ORGANIZATION_BLOCK OB 1
	VAR_TEMP
		TMPDUMMY	: INT;
		DTTEMP		: DATE_AND_TIME;
	END_VAR
BEGIN

	// Check forwarding of compound data type to FC
	// (This will create implicit DB pointers)
	AUF		DB 42
	LAR1		P##DTTEMP
	L		DW#16#12345678
	T		D [AR1, P#0.0]
	L		DW#16#87654321
	T		DBD 4
	L		DW#16#AABBCCDD
	T		D [AR1, P#4.0]
	L		DW#16#DDCCBBAA
	T		DBD 8
	CALL		FC 1 (
		DTTEMP	:= #DTTEMP,
		DTDB	:= DB42.DTVAR,
	)

	// Check forwarding of compound data type from FB to FC
	CALL		FB 10, DB 10 (
		DUMMYIN	:= 42,
		DTVAR	:= DB42.DTVAR,
	)


	CALL SFC 46 // STOP CPU
END_ORGANIZATION_BLOCK


FUNCTION FC 1 : VOID
	VAR_INPUT
		DTTEMP		: DATE_AND_TIME;
		DTDB		: DATE_AND_TIME;
	END_VAR
	VAR_TEMP
		DBNR		: INT;
	END_VAR
BEGIN
	// Load #DTTEMP into AR1
	L		P##DTTEMP
	LAR1
	UD		DW#16#FF000000
	__ASSERT==	__ACCU 1,	DW#16#87000000
	// Check the DB-pointer pointed to by #DTTEMP
	L		W [AR1, P#0.0]
	__ASSERT==	__ACCU 1,	0 // DB-nr
	T		#DBNR
	L		D [AR1, P#2.0]
	__ASSERT==	__ACCU 1,	DW#16#87000010
	LAR2
	AUF		DB [#DBNR]
	// Check the actual values
	L		D [AR2, P#0.0]
	__ASSERT==	__ACCU 1,	DW#16#12345678
	L		D [AR2, P#4.0]
	__ASSERT==	__ACCU 1,	DW#16#AABBCCDD


	// Load #DTDB into AR1
	L		P##DTDB
	LAR1
	UD		DW#16#FF000000
	__ASSERT==	__ACCU 1,	DW#16#87000000
	// Check the DB-pointer pointed to by #DTDB
	L		W [AR1, P#0.0]
	__ASSERT==	__ACCU 1,	42 // DB-nr
	T		#DBNR
	L		D [AR1, P#2.0]
	__ASSERT==	__ACCU 1,	DW#16#84000020
	LAR2
	AUF		DB [#DBNR]
	// Check the actual values
	L		D [AR2, P#0.0]
	__ASSERT==	__ACCU 1,	DW#16#87654321
	L		D [AR2, P#4.0]
	__ASSERT==	__ACCU 1,	DW#16#DDCCBBAA
END_FUNCTION


FUNCTION_BLOCK FB 10
	VAR_INPUT
		DUMMYIN		: INT;
		DTVAR		: DATE_AND_TIME;
	END_VAR
BEGIN
	CALL FC 11 (
		DTIN	:= #DTVAR,
	)
END_FUNCTION_BLOCK


FUNCTION FC 11 : VOID
	VAR_INPUT
		DTIN		: DATE_AND_TIME;
	END_VAR
	VAR_TEMP
		DBNR		: INT;
	END_VAR
BEGIN
	// Load #DTDB into AR1
	L		P##DTIN
	LAR1
	UD		DW#16#FF000000
	__ASSERT==	__ACCU 1,	DW#16#87000000
	// Check the DB-pointer pointed to by #DTIN
	L		W [AR1, P#0.0]
	__ASSERT==	__ACCU 1,	10 // DB-nr
	T		#DBNR
	L		D [AR1, P#2.0]
	__ASSERT==	__ACCU 1,	DW#16#84000010
	LAR2
	AUF		DB [#DBNR]
	// Check the actual values
	L		D [AR2, P#0.0]
	__ASSERT==	__ACCU 1,	DW#16#87654321
	L		D [AR2, P#4.0]
	__ASSERT==	__ACCU 1,	DW#16#DDCCBBAA
END_FUNCTION


DATA_BLOCK DB 10
	FB 10
BEGIN
END_DATA_BLOCK


DATA_BLOCK DB 42
	STRUCT
		DUMMY1		: INT;
		DUMMY2		: INT;
		DTVAR		: DATE_AND_TIME;
		DUMMY3		: INT;
	END_STRUCT;
BEGIN
END_DATA_BLOCK
